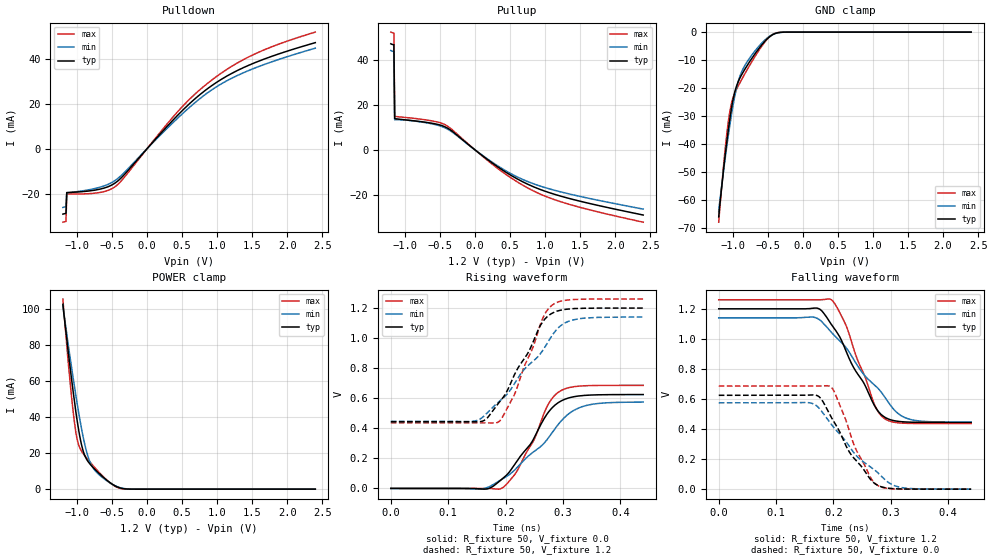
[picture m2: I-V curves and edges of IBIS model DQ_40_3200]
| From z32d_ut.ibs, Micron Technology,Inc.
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| MODEL DQ_40_3200 (40 Ohm Data I/O with no ODT, 1600-3200Mbps)
[Model]   DQ_40_3200
Model_type   I/O
Vinl = 905.000mV
Vinh = 1015.000mV
Vmeas = 960.000mV
Vref = 1200.000mV
Cref = 0.0pF
Rref = 50.000Ohm
|   typ   min   max
|C_comp   0.636pF   0.586pF   0.686pF
C_comp_pullup   0.318pF   0.293pF   0.343pF
C_comp_pulldown   0.318pF   0.293pF   0.343pF
[Model Spec]
| Timing spec test load voltage corners
Vref   1.2000V   1.1400V   1.2600V
| Dynamic Overshoot Parameters from DDR4 Specification
|D_overshoot_ampl_h   0.40   NA   NA
|D_overshoot_ampl_l   0.40   NA   NA
|D_overshoot_area_h   0.0800n   NA   NA
|D_overshoot_area_l   0.0800n   NA   NA
[Voltage Range]   1.2000V   1.1400V   1.2600V
| Junction Temperature (Ambient temp is 35C typ, 125C min, -40C max)
[Temperature Range]   50.0   140.0   -40.0
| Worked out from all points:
|   slope of the pulldown table from 0 to 0.18 V, typ, clamps not added: 28.6 ohm
|   slope of the pullup table from 0 to 0.18 V, typ, clamps not added: 41.6 ohm
|   GND clamp passes 1 mA (typ) near -0.44 V on its own axis
|   POWER clamp passes 1 mA (typ) near -0.41 V on its own axis
|   rising waveform, R_fixture 50, V_fixture 0.0: 20-80 % time 63.6ps typ, 85.8ps min, 49.8ps max; typ from 0 V to 0.625 V
|   rising waveform, R_fixture 50, V_fixture 1.2: 20-80 % time 62.3ps typ, 87.2ps min, 48.6ps max; typ from 0.444 V to 1.2 V
|   falling waveform, R_fixture 50, V_fixture 1.2: 20-80 % time 61.1ps typ, 87.4ps min, 46.3ps max; typ from 1.2 V to 0.444 V
|   falling waveform, R_fixture 50, V_fixture 0.0: 20-80 % time 60.7ps typ, 85.3ps min, 45.1ps max; typ from 0.625 V to 0 V
[Pulldown]
|   Voltage   I(typ)   I(min)   I(max)
-1.2V     -29.12mA   -26.14mA   -32.71mA
-1.156V   -28.8mA    -25.82mA   -32.39mA
-1.145V   -19.51mA   -19.63mA   -20.16mA
-687.3mV  -18.1mA    -17.28mA   -19.55mA
-447.3mV  -15.08mA   -13.94mA   -16.69mA
-338.2mV  -11.99mA   -11.02mA   -13.27mA
469.1mV   15.9mA     14.55mA    17.58mA
698.2mV   22.62mA    20.88mA    24.73mA
938.2mV   28.41mA    26.51mA    30.92mA
1.222V    33.76mA    31.6mA     36.95mA
1.516V    38.02mA    35.66mA    41.88mA
2.4V      47.23mA    44.77mA    51.93mA
[GND Clamp]
|   Voltage   I(typ)   I(min)   I(max)
-1.2V     -66.16mA   -64.28mA   -68.09mA
-1.135V   -50.09mA   -50.4mA    -48.84mA
-1.091V   -40.55mA   -42.05mA   -37.85mA
-1.047V   -32.05mA   -34.3mA    -29.3mA
-1.004V   -25.21mA   -27.36mA   -24.13mA
-970.9mV  -21.44mA   -22.9mA    -21.89mA
-927.3mV  -18.1mA    -18.21mA   -19.59mA
-840mV    -13.84mA   -12.53mA   -15.5mA
-632.7mV  -6.061mA   -5.231mA   -6.759mA
-447.3mV  -1.181mA   -1.089mA   -1.122mA
-250.9mV  -9.403uA   -28.92uA   310.9nA
2.4V      0A         0A         0A
[Pullup]
|   Voltage   I(typ)   I(min)   I(max)
-1.2V     47.33mA    44.35mA    52.54mA
-1.156V   46.84mA    43.82mA    52.08mA
-1.145V   13.94mA    13.44mA    14.91mA
-741.8mV  12.46mA    12.31mA    13.54mA
-425.5mV  10.24mA    9.779mA    11.21mA
-327.3mV  8.361mA    7.97mA     9.047mA
98.18mV   -2.398mA   -2.268mA   -2.609mA
403.6mV   -9.233mA   -8.673mA   -10.12mA
676.4mV   -14.17mA   -13.15mA   -15.66mA
960mV     -18.01mA   -16.46mA   -20.13mA
1.462V    -22.63mA   -20.52mA   -25.34mA
2.4V      -29.08mA   -26.44mA   -32.28mA
[POWER Clamp]
|   Voltage   I(typ)   I(min)   I(max)
-1.2V     102.5mA    102mA      105.3mA
-1.135V   79.77mA    83.1mA     75.19mA
-1.069V   58.73mA    65.56mA    48.42mA
-1.015V   42.78mA    51.76mA    31.4mA
-981.8mV  34.36mA    43.96mA    25.35mA
-905.5mV  20.47mA    27.86mA    19.42mA
-850.9mV  15.87mA    19.19mA    16.74mA
-807.3mV  13.63mA    14.47mA    14.72mA
-709.1mV  9.665mA    8.957mA    10.4mA
-501.8mV  2.908mA    2.849mA    2.742mA
-250.9mV  22.56uA    71.67uA    -929.3nA
2.4V      0A         0A         0A
[Ramp]
|   typ   min   max
| 20% - 80%
dV/dt_r   374.75m/63.58p   344.61m/85.76p   411.51m/49.80p
dV/dt_f   453.55m/61.15p   416.27m/87.34p   494.02m/46.29p
| Slew rate: Power terminated
|SR_r[V/ns]   7.28   4.77   10.18
|SR_f[V/ns]   7.42   4.77   10.67
| 25% - 75%
|dV/dt_r   312.29m/52.61p   287.17m/71.67p   342.92m/41.18p
|dV/dt_f   377.96m/50.69p   346.89m/71.76p   411.68m/38.60p
| Slew rate: Power terminated
|SR_r[V/ns]   7.36   4.83   10.29
|SR_f[V/ns]   7.46   4.83   10.67
R_load = 50
[Rising Waveform]
R_fixture = 50
V_fixture = 0.0
|   Time   V(typ)   V(min)   V(max)
0s        6.048uV    34.79uV    354.8nV
165ps     -4.693mV   1.799mV    267.7uV
192ps     56.09mV    56.94mV    -1.218mV
220ps     183mV      138.5mV    115.4mV
250ps     337mV      246.8mV    326.1mV
273ps     498.3mV    327.5mV    549.3mV
292ps     570.9mV    426.4mV    639.7mV
314ps     606mV      507.1mV    673.5mV
340ps     619.5mV    551mV      683.3mV
440ps     624.6mV    574.4mV    685.8mV
[Rising Waveform]
R_fixture   = 50
V_fixture   = 1.2
V_fixture_min = 1.14
V_fixture_max = 1.26
|   Time   V(typ)   V(min)   V(max)
0s        444.1mV    446.1mV    436.6mV
157ps     445mV      465.2mV    436.7mV
187ps     563.5mV    571.9mV    440.8mV
215ps     752.6mV    693.9mV    620.5mV
240ps     907.8mV    820.2mV    872.8mV
264ps     1.104V     913.1mV    1.125V
280ps     1.163V     1.012V     1.216V
299ps     1.188V     1.091V     1.248V
320ps     1.197V     1.123V     1.257V
440ps     1.2V       1.14V      1.26V
[Falling Waveform]
R_fixture   = 50
V_fixture   = 1.2
V_fixture_min = 1.14
V_fixture_max = 1.26
|   Time   V(typ)   V(min)   V(max)
0s        1.2V       1.14V      1.26V
171ps     1.205V     1.138V     1.26V
195ps     1.104V     1.05V      1.263V
220ps     936.8mV    951.3mV    1.107V
249ps     730.4mV    781.9mV    799.2mV
270ps     566.7mV    698.7mV    576.6mV
286ps     487.8mV    631.7mV    478.6mV
309ps     453.4mV    515.7mV    443.3mV
330ps     446.4mV    468.4mV    437.9mV
440ps     444.1mV    446.2mV    436.6mV
[Falling Waveform]
R_fixture = 50
V_fixture = 0.0
|   Time   V(typ)   V(min)   V(max)
0s        624.6mV    574.7mV    685.9mV
169ps     625.5mV    559.5mV    685.8mV
179ps     598.2mV    520.8mV    686.9mV
193ps     500.6mV    446.6mV    685.8mV
203ps     434.8mV    400.5mV    635mV
229ps     239.7mV    277.4mV    371.7mV
241ps     184.3mV    218.1mV    251.2mV
275ps     29.84mV    117.6mV    30.16mV
318ps     1.206mV    11.37mV    600.4uV
440ps     6.181uV    43.58uV    369nV
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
